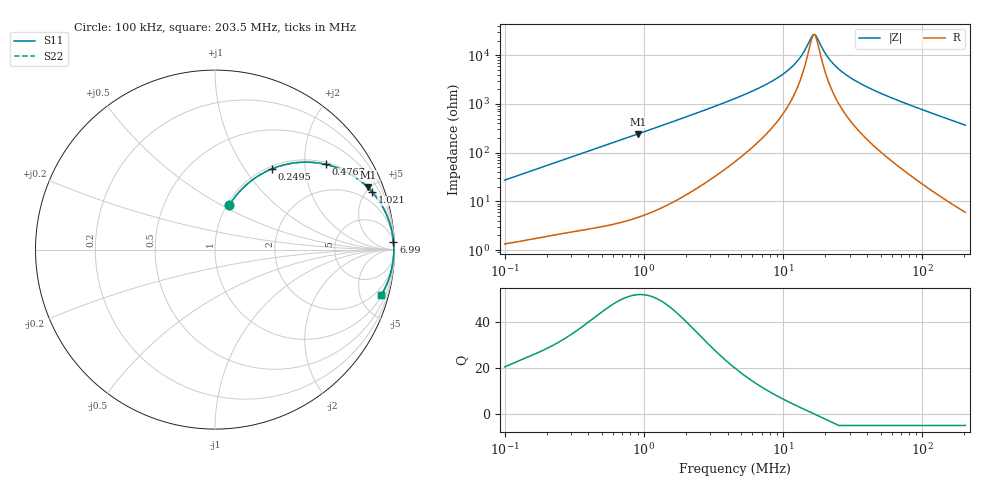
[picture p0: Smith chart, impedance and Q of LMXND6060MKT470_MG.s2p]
! LMXND6060MKT470_MG  S-PARAMETER MODEL  ( General Type )
! Model Generated by TAIYO YUDEN Corporation (https://www.yuden.co.jp/en/)
! Version 1.0
! TAIYO YUDEN Control No. 191025NI43SB-FBB
! Copyright(c) 2019 TAIYO YUDEN CO.,LTD. All Rights Reserved.
! Product Description (link to TY-COMPAS)
! https://ds.yuden.co.jp/TYCOMPAS/or/detail?pn=LMXND6060MKT470MMG&u=M
! Products Name : Inductors
! Characteristics :
!  Inductance : 47 uH , SRF(min) : 6.0 MHz , DC Resistance(max) : 1.158 Ohm
!  Rated Current : Saturation :520 mA , Temp Rise : 460 mA (40 degC)
!  Case Size : 6.0 x 6.0 / 0.236 x 0.236 [mm/inch] , Thickness : 1.2 / 0.047 [mm/inch]
!  (Conditions: Temperature = 25 degC , DC Bias Current/Voltage = 0A / 0V)
! External Node Assignments :
!  1  o---GGG---o  2
! GND o---------o GND
! Frequency Range : 0.1MHz  -  203.457813MHz  [ 402 STEP ]
# MHz S RI R 50
! Freq[MHz].  S11 Real  S11 Imag  S21 Real  S21 Imag  S12 Real  S12 Imag  S22 Real  S22 Imag
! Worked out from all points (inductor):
!   401 points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, 100 kHz to 203.5 MHz, reference 50 ohm
!   read as one part in series: L = 43.3 uH near 103.9 kHz
!   highest Q = 51.6 at 910.9 kHz (marker M1), where L = 42.5 uH
!   self-resonance near 16.47 MHz
!   S11 on the Smith chart (normalised r, x): 100 kHz: 1.03, +0.55; 249.5 kHz: 1.04, +1.34; 476.7 kHz: 1.06, +2.55; 1.021 MHz: 1.11, +5.46; 6.99 MHz: 5, +45; 203.5 MHz: 1.12, -7.32
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0.1  0.0798 0.2476  0.9202 -0.2476  0.9202 -0.2476  0.0798 0.2476
0.160983  0.1695 0.3562  0.8305 -0.3562  0.8305 -0.3562  0.1695 0.3562
0.249469  0.3165 0.4494  0.6835 -0.4494  0.6835 -0.4494  0.3165 0.4494
0.358236  0.4804 0.4865  0.5196 -0.4865  0.5196 -0.4865  0.4804 0.4865
0.476691  0.6166 0.4748  0.3834 -0.4748  0.3834 -0.4748  0.6166 0.4748
0.910872  0.8508 0.3467  0.1492 -0.3467  0.1492 -0.3467  0.8508 0.3467
1.021139  0.877 0.3189  0.123 -0.3189  0.123 -0.3189  0.877 0.3189
1.283332  0.9174 0.2653  0.0826 -0.2653  0.0826 -0.2653  0.9174 0.2653
2.316038  0.9713 0.1538  0.0287 -0.1538  0.0287 -0.1538  0.9713 0.1538
4.51063  0.9903 0.0762  0.00974 -0.0762  0.00974 -0.0762  0.9903 0.0762
6.989956  0.9943 0.0439  0.00572 -0.0439  0.00572 -0.0439  0.9943 0.0439
9.480111  0.9955 0.0266  0.00446 -0.0266  0.00446 -0.0266  0.9955 0.0266
11.68952  0.996 0.0162  0.004 -0.0162  0.004 -0.0162  0.996 0.0162
13.61338  0.9962 0.00914  0.00381 -0.00914  0.00381 -0.00914  0.9962 0.00914
16.15871  0.9963 0.00142  0.00373 -0.00142  0.00373 -0.00142  0.9963 0.00142
17.10883  0.9963 -0.00114  0.00373 0.00114  0.00373 0.00114  0.9963 -0.00114
21.09615  0.9962 -0.0106  0.00384 0.0106  0.00384 0.0106  0.9962 -0.0106
26.51291  0.9958 -0.0215  0.00419 0.0215  0.00419 0.0215  0.9958 -0.0215
36.64946  0.9947 -0.0389  0.00526 0.0389  0.00526 0.0389  0.9947 -0.0389
57.88634  0.9912 -0.0708  0.00882 0.0708  0.00882 0.0708  0.9912 -0.0708
110.6105  0.9754 -0.1419  0.0246 0.1419  0.0246 0.1419  0.9754 -0.1419
203.4578  0.9271 -0.252  0.0729 0.252  0.0729 0.252  0.9271 -0.252
